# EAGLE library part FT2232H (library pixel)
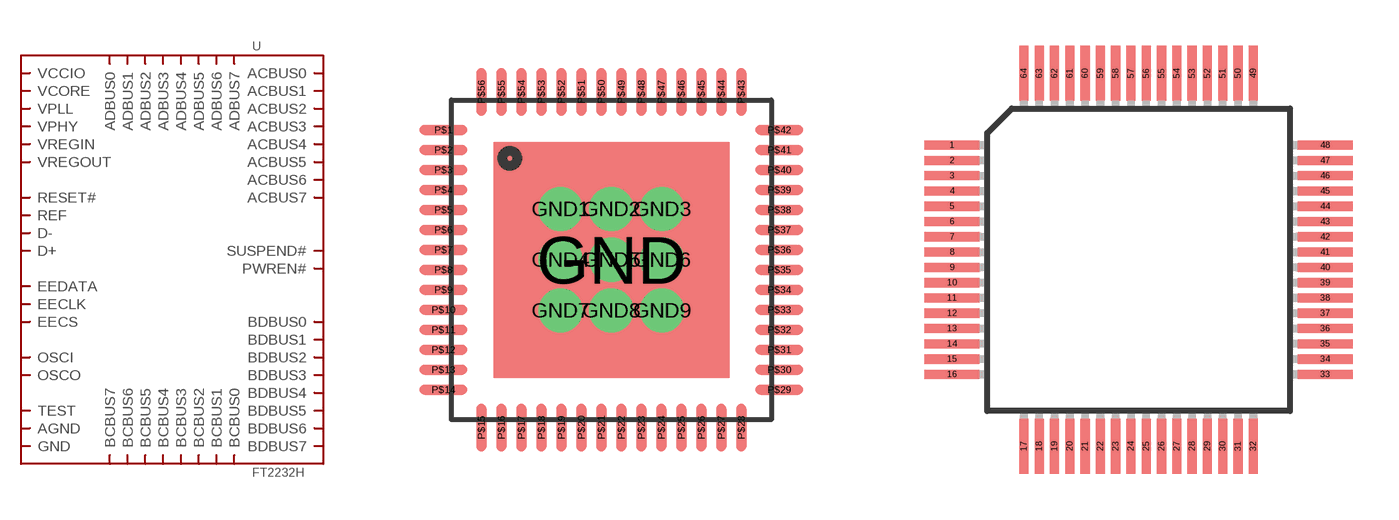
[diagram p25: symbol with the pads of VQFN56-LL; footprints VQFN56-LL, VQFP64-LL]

Designator prefix -

## FT2232HVQFN56-LL  [VQFN56-LL]
GND  GND
GND1  GND
GND2  GND
GND3  GND
GND4  GND
GND5  AGND
GND6  GND
GND7  GND
GND8  GND
GND9  GND
P$1  EECS
P$2  VCORE
P$3  OSCI
P$4  OSCO
P$5  VPHY
P$6  REF
P$7  D-
P$8  D+
P$9  VPLL
P$10  TEST
P$11  RESET#
P$12  ADBUS0
P$13  ADBUS1
P$14  ADBUS2
P$15  ADBUS3
P$16  VCCIO
P$17  ADBUS4
P$18  ADBUS5
P$19  ADBUS6
P$20  ADBUS7
P$21  GND
P$22  ACBUS0
P$23  ACBUS1
P$24  ACBUS2
P$25  ACBUS3
P$26  ACBUS4
P$27  ACBUS5
P$28  ACBUS6
P$29  ACBUS7
P$30  SUSPEND#
P$31  VCORE
P$32  BDBUS0
P$33  BDBUS1
P$34  BDBUS2
P$35  BDBUS3
P$36  VCCIO
P$37  BDBUS4
P$38  BDBUS5
P$39  BDBUS6
P$40  BDBUS7
P$41  GND
P$42  BCBUS0
P$43  VREGOUT
P$44  VREGIN
P$45  GND
P$46  BCBUS1
P$47  BCBUS2
P$48  BCBUS3
P$49  BCBUS4
P$50  VCCIO
P$51  BCBUS5
P$52  BCBUS6
P$53  BCBUS7
P$54  PWREN#
P$55  EEDATA
P$56  EECLK

## FT2232HVQFP64-LL  [VQFP64-LL]
1  GND
2  OSCI
3  OSCO
4  VPHY
5  GND
6  REF
7  D-
8  D+
9  VPLL
10  AGND
11  GND
12  VCORE
13  TEST
14  RESET#
15  GND
16  ADBUS0
17  ADBUS1
18  ADBUS2
19  ADBUS3
20  VCCIO
21  ADBUS4
22  ADBUS5
23  ADBUS6
24  ADBUS7
25  GND
26  ACBUS0
27  ACBUS1
28  ACBUS2
29  ACBUS3
30  ACBUS4
31  VCCIO
32  ACBUS5
33  ACBUS6
34  ACBUS7
35  GND
36  SUSPEND#
37  VCORE
38  BDBUS0
39  BDBUS1
40  BDBUS2
41  BDBUS3
42  VCCIO
43  BDBUS4
44  BDBUS5
45  BDBUS6
46  BDBUS7
47  GND
48  BCBUS0
49  VREGOUT
50  VREGIN
51  GND
52  BCBUS1
53  BCBUS2
54  BCBUS3
55  BCBUS4
56  VCCIO
57  BCBUS5
58  BCBUS6
59  BCBUS7
60  PWREN#
61  EEDATA
62  EECLK
63  EECS
64  VCORE

## FT2232HVQFP64  [VQFP64]
Pads as for VQFP64-LL

## Footprint VQFN56-LL (pad centres in mm)
smd 5.9 x 5.9: GND 0,0
drill 0.6: GND1 -1.27,1.27; GND2 0,1.27; GND3 1.27,1.27; GND4 -1.27,0; GND5 0,0; GND6 1.27,0; GND7 -1.27,-1.27; GND8 0,-1.27; GND9 1.27,-1.27
smd 1.2 x 0.25: P$1 -4.2,3.25; P$2 -4.2,2.75; P$3 -4.2,2.25; P$4 -4.2,1.75; P$5 -4.2,1.25; P$6 -4.2,0.75; P$7 -4.2,0.25; P$8 -4.2,-0.25; P$9 -4.2,-0.75; P$10 -4.2,-1.25; P$11 -4.2,-1.75; P$12 -4.2,-2.25; P$13 -4.2,-2.75; P$14 -4.2,-3.25; P$29 4.2,-3.25; P$30 4.2,-2.75; P$31 4.2,-2.25; P$32 4.2,-1.75; P$33 4.2,-1.25; P$34 4.2,-0.75; P$35 4.2,-0.25; P$36 4.2,0.25; P$37 4.2,0.75; P$38 4.2,1.25; P$39 4.2,1.75; P$40 4.2,2.25; P$41 4.2,2.75; P$42 4.2,3.25
smd 0.25 x 1.2: P$15 -3.25,-4.2; P$16 -2.75,-4.2; P$17 -2.25,-4.2; P$18 -1.75,-4.2; P$19 -1.25,-4.2; P$20 -0.75,-4.2; P$21 -0.25,-4.2; P$22 0.25,-4.2; P$23 0.75,-4.2; P$24 1.25,-4.2; P$25 1.75,-4.2; P$26 2.25,-4.2; P$27 2.75,-4.2; P$28 3.25,-4.2; P$43 3.25,4.2; P$44 2.75,4.2; P$45 2.25,4.2; P$46 1.75,4.2; P$47 1.25,4.2; P$48 0.75,4.2; P$49 0.25,4.2; P$50 -0.25,4.2; P$51 -0.75,4.2; P$52 -1.25,4.2; P$53 -1.75,4.2; P$54 -2.25,4.2; P$55 -2.75,4.2; P$56 -3.25,4.2

## Footprint VQFP64-LL (pad centres in mm)
64-lead VQVP Source. http://www.atmel.com/dyn/resources/prod_documents/doc4136.pdf
smd 1.8 x 0.3: 1 -6.1,3.75; 2 -6.1,3.25; 3 -6.1,2.75; 4 -6.1,2.25; 5 -6.1,1.75; 6 -6.1,1.25; 7 -6.1,0.75; 8 -6.1,0.25; 9 -6.1,-0.25; 10 -6.1,-0.75; 11 -6.1,-1.25; 12 -6.1,-1.75; 13 -6.1,-2.25; 14 -6.1,-2.75; 15 -6.1,-3.25; 16 -6.1,-3.75; 33 6.1,-3.75; 34 6.1,-3.25; 35 6.1,-2.75; 36 6.1,-2.25; 37 6.1,-1.75; 38 6.1,-1.25; 39 6.1,-0.75; 40 6.1,-0.25; 41 6.1,0.25; 42 6.1,0.75; 43 6.1,1.25; 44 6.1,1.75; 45 6.1,2.25; 46 6.1,2.75; 47 6.1,3.25; 48 6.1,3.75
smd 0.3 x 1.8: 17 -3.75,-6.1; 18 -3.25,-6.1; 19 -2.75,-6.1; 20 -2.25,-6.1; 21 -1.75,-6.1; 22 -1.25,-6.1; 23 -0.75,-6.1; 24 -0.25,-6.1; 25 0.25,-6.1; 26 0.75,-6.1; 27 1.25,-6.1; 28 1.75,-6.1; 29 2.25,-6.1; 30 2.75,-6.1; 31 3.25,-6.1; 32 3.75,-6.1; 49 3.75,6.1; 50 3.25,6.1; 51 2.75,6.1; 52 2.25,6.1; 53 1.75,6.1; 54 1.25,6.1; 55 0.75,6.1; 56 0.25,6.1; 57 -0.25,6.1; 58 -0.75,6.1; 59 -1.25,6.1; 60 -1.75,6.1; 61 -2.25,6.1; 62 -2.75,6.1; 63 -3.25,6.1; 64 -3.75,6.1

## Footprint VQFP64 (pad centres in mm)
64-lead VQVP Source. http://www.atmel.com/dyn/resources/prod_documents/doc4136.pdf
smd 1 x 0.3: 1 -5.7,3.75; 2 -5.7,3.25; 3 -5.7,2.75; 4 -5.7,2.25; 5 -5.7,1.75; 6 -5.7,1.25; 7 -5.7,0.75; 8 -5.7,0.25; 9 -5.7,-0.25; 10 -5.7,-0.75; 11 -5.7,-1.25; 12 -5.7,-1.75; 13 -5.7,-2.25; 14 -5.7,-2.75; 15 -5.7,-3.25; 16 -5.7,-3.75; 33 5.7,-3.75; 34 5.7,-3.25; 35 5.7,-2.75; 36 5.7,-2.25; 37 5.7,-1.75; 38 5.7,-1.25; 39 5.7,-0.75; 40 5.7,-0.25; 41 5.7,0.25; 42 5.7,0.75; 43 5.7,1.25; 44 5.7,1.75; 45 5.7,2.25; 46 5.7,2.75; 47 5.7,3.25; 48 5.7,3.75
smd 0.3 x 1: 17 -3.75,-5.7; 18 -3.25,-5.7; 19 -2.75,-5.7; 20 -2.25,-5.7; 21 -1.75,-5.7; 22 -1.25,-5.7; 23 -0.75,-5.7; 24 -0.25,-5.7; 25 0.25,-5.7; 26 0.75,-5.7; 27 1.25,-5.7; 28 1.75,-5.7; 29 2.25,-5.7; 30 2.75,-5.7; 31 3.25,-5.7; 32 3.75,-5.7; 49 3.75,5.7; 50 3.25,5.7; 51 2.75,5.7; 52 2.25,5.7; 53 1.75,5.7; 54 1.25,5.7; 55 0.75,5.7; 56 0.25,5.7; 57 -0.25,5.7; 58 -0.75,5.7; 59 -1.25,5.7; 60 -1.75,5.7; 61 -2.25,5.7; 62 -2.75,5.7; 63 -3.25,5.7; 64 -3.75,5.7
